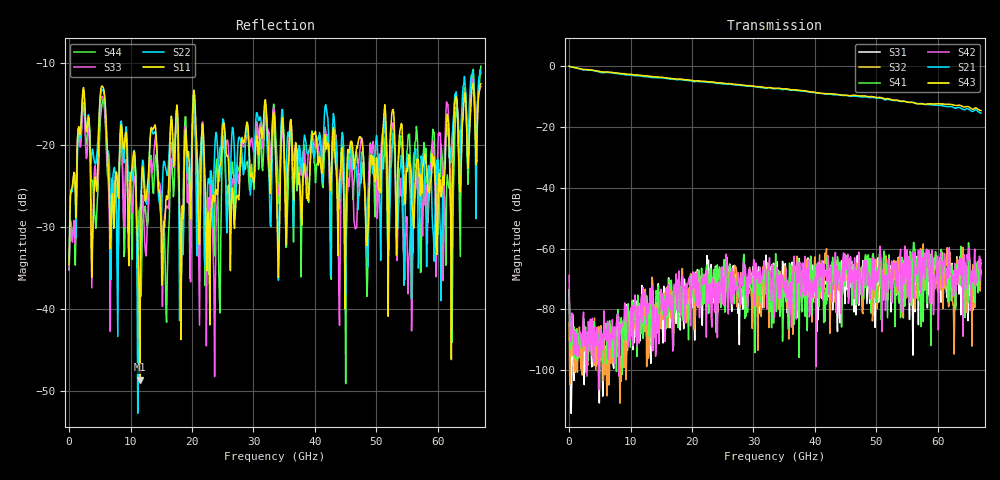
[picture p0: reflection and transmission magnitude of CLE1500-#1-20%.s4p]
!Keysight Technologies,N5247B,US50470101,A.16.20.02
!Date: Thursday, March 13, 2025 10:13:18
!Correction: S11(C  4-Port  )
!S12(C  4-Port  )
!S13(C  4-Port  )
!S14(C  4-Port  )
!S21(C  4-Port  )
!S22(C  4-Port  )
!S23(C  4-Port  )
!S24(C  4-Port  )
!S31(C  4-Port  )
!S32(C  4-Port  )
!S33(C  4-Port  )
!S34(C  4-Port  )
!S41(C  4-Port  )
!S42(C  4-Port  )
!S43(C  4-Port  )
!S44(C  4-Port  )
!S4P File: Measurements: <S11,S12,S13,S14>,
!<S21,S22,S23,S24>,
!<S31,S32,S33,S34>,
!<S41,S42,S43,S44>:
# Hz S  dB  R 50
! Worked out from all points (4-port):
!   601 points, 10 MHz to 67 GHz, reference 50 ohm
!   strongest paths, dB at 10 MHz, 16.76 GHz, 33.51 GHz, 50.25 GHz, 67 GHz:
!     S43: 0.0, -4.1, -7.3, -10.3, -14.6
!     S21: 0.0, -4.3, -7.4, -10.5, -15.4
!     S42: -68.7, -79.6, -76.1, -70.5, -63.5
!     S41: -73.6, -75.4, -71.0, -70.6, -68.2
!     S32: -84.3, -74.3, -70.4, -74.4, -67.1
!     S31: -73.5, -74.8, -68.6, -63.0, -64.7
!   lowest |S11| = -48.6 dB at 11.51 GHz (marker M1), VSWR 1.01, Z = 50.1 + j0.366 ohm
!   |S11| at or under -10 dB: start of sweep to end of sweep
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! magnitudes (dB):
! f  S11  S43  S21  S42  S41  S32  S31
! 10 MHz  -34.5  0.0  0.0  -68.7  -73.6  -84.3  -73.5
! 5.481 GHz  -12.8  -1.9  -2.1  -91.5  -97.5  -92.5  -108.5
! 11.51 GHz  -48.6  -3.0  -3.2  -82.8  -83.1  -82.6  -90.4
! 13.63 GHz  -18.1  -3.4  -3.7  -93.6  -79.1  -71.7  -80.5
! 32.05 GHz  -15.2  -7.1  -7.2  -72.5  -72.1  -67.6  -62.1
! 55.5 GHz  -22.2  -11.9  -11.9  -76.1  -60.8  -64.5  -67.5
! 67 GHz  -12.5  -14.6  -15.4  -63.5  -68.2  -67.1  -64.7
